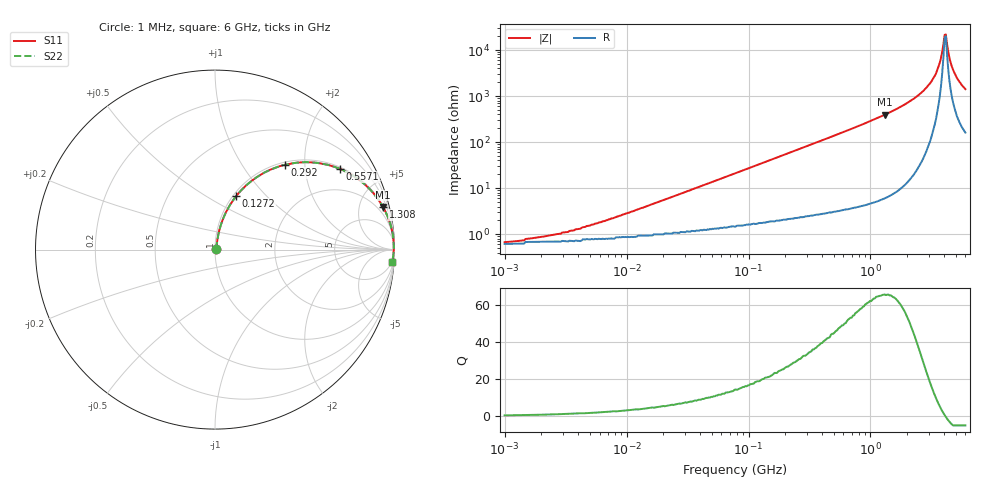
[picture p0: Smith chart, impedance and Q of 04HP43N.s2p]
# MHz S MA R 50
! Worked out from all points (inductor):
!   378 points, 1 MHz to 6 GHz, reference 50 ohm
!   read as one part in series: L = 43 nH near 9.821 MHz
!   highest Q = 65.4 at 1.308 GHz (marker M1), where L = 48 nH
!   self-resonance near 4.053 GHz
!   S11 on the Smith chart (normalised r, x): 1 MHz: 1.01, +0.01; 127.2 MHz: 1.04, +0.69; 292 MHz: 1.05, +1.58; 557.1 MHz: 1.06, +3.07; 1.308 GHz: 1.11, +7.87; 6 GHz: 4, -28
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1  0.006812 23.1  0.994 -0.2  0.994 -0.2  0.006812 23.1
2.891  0.01 47.4  0.993 -0.4  0.993 -0.4  0.01 47.4
4.279  0.014 56.5  0.993 -0.7  0.993 -0.7  0.014 56.5
18.312  0.05 75.9  0.989 -2.8  0.989 -2.8  0.05 75.9
78.359  0.205 74.2  0.965 -11.8  0.965 -11.8  0.205 74.2
127.216  0.321 68.4  0.931 -18.7  0.931 -18.7  0.321 68.4
291.957  0.612 50.5  0.772 -37.7  0.772 -37.7  0.612 50.5
335.312  0.665 46.7  0.729 -41.6  0.729 -41.6  0.665 46.7
557.089  0.83 32.7  0.541 -56.1  0.541 -56.1  0.83 32.7
1308.351  0.966 14.2  0.245 -74.9  0.245 -74.9  0.966 14.2
1434.864  0.972 12.7  0.22 -76.4  0.22 -76.4  0.972 12.7
2276.372  0.991 6.4  0.112 -82.3  0.112 -82.3  0.991 6.4
3144.458  0.996 2.8  0.049 -83.7  0.049 -83.7  0.996 2.8
3448.517  0.996 1.8  0.032 -82.3  0.032 -82.3  0.996 1.8
3695.704  0.996 1.1  0.019 -78.2  0.019 -78.2  0.996 1.1
3870.263  0.996 0.6  0.011 -69.7  0.011 -69.7  0.996 0.6
4053.066  0.996 0.1  0.00467 -29.5  0.00467 -29.5  0.996 0.1
4147.681  0.996 -0.1  0.00458 23.4  0.00458 23.4  0.996 -0.1
4343.587  0.995 -0.6  0.011 65.3  0.011 65.3  0.995 -0.6
4654.933  0.995 -1.3  0.023 76.1  0.023 76.1  0.995 -1.3
5105.049  0.993 -2.2  0.04 79.2  0.04 79.2  0.993 -2.2
6000  0.99 -4.0  0.07 79.5  0.07 79.5  0.99 -4.0
